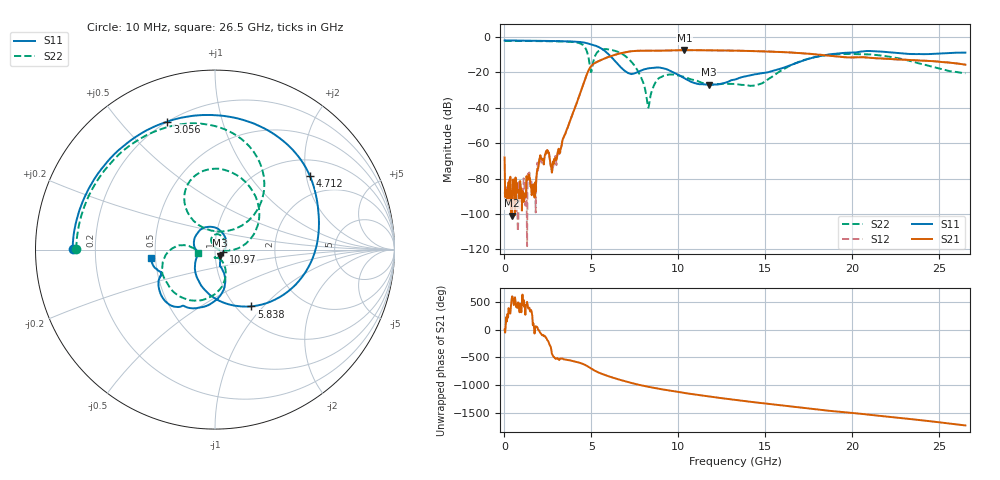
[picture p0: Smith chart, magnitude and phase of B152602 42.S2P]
!  2-Port S-parameters saved by WinCal
! VAR MeasName=S-Parameters (CALIBRATED_DATA) read from VNA (N5242A)
! VAR MeasDate=2016-1-5 16:32:14
! VAR NAME=B152602 42
! VAR FILENAME=B152602 42.S2P
! VAR DATE=2016-1-5 16:32:14
! VAR PHYS_PORTS=1,2
# Hz S DB R 50
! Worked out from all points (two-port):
!   801 points, 10 MHz to 26.5 GHz, reference 50 ohm
!   highest |S21| = -7.47 dB at 10.34 GHz (marker M1); lowest = -100.9 dB at 440.5 MHz (marker M2)
!   |S21| within 3 dB of the highest: 6.238 GHz to 18.54 GHz (12.3 GHz wide, 99.3 % of centre)
!   lowest |S11| = -27.1 dB at 11.73 GHz (marker M3), VSWR 1.09, Z = 52.9 - j3.53 ohm
!   |S11| at or under -10 dB: 6.005 GHz to 18.63 GHz (12.62 GHz wide, 102 % of centre)
!   |S22| runs from -39.9 to -2.2 dB; largest |S21 - S12| = 0.0031
!   S11 on the Smith chart (normalised r, x): 10 MHz: 0.12, +0.00; 3.056 GHz: 0.20, +0.68; 4.712 GHz: 1.41, +2.10; 5.838 GHz: 1.17, -0.86; 10.97 GHz: 1.10, -0.03; 26.5 GHz: 0.47, -0.05
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1e7  -2.01 179.7  -68.07 0.8  -88.54 20.5  -2.23 179.8
4.404625e8  -2.04 170.9  -100.94 -124.4  -86.64 126.1  -2.25 173.2
1.698738e9  -2.20 144.7  -84.91 45.0  -89.84 24.8  -2.36 153.3
2.427212e9  -2.28 127.7  -65.81 -160.7  -64.42 -162.4  -2.44 140.5
2.758338e9  -2.32 118.9  -72.60 -89.8  -76.01 -110.0  -2.47 134.0
3.05635e9  -2.37 110.4  -65.44 -151.4  -66.65 -154.8  -2.53 127.5
4.447075e9  -3.00 54.0  -29.22 112.2  -29.24 112.3  -4.14 74.1
4.711975e9  -3.49 37.9  -21.80 74.6  -21.82 74.8  -7.47 49.9
5.009988e9  -4.31 18.4  -16.24 15.7  -16.25 15.9  -19.29 101.8
5.8378e9  -8.50 -57.3  -11.89 -100.6  -11.86 -100.6  -6.92 87.6
6.6325e9  -16.60 -139.2  -9.35 -179.4  -9.34 -179.5  -8.93 48.8
7.360975e9  -20.89 -169.4  -8.03 118.4  -8.03 118.4  -14.76 12.5
8.255012e9  -17.81 154.1  -7.83 55.3  -7.82 55.2  -39.82 42.9
8.851038e9  -17.25 120.0  -7.83 20.7  -7.84 20.6  -23.57 107.9
1.03411e10  -23.31 21.8  -7.47 -55.6  -7.47 -55.6  -22.63 45.6
1.097024e10  -26.16 -16.4  -7.50 -85.0  -7.49 -84.9  -24.52 15.6
1.173182e10  -27.06 -48.8  -7.57 -118.2  -7.56 -118.1  -26.71 -27.7
1.3255e10  -24.04 -63.1  -7.78 -179.8  -7.78 -179.8  -26.55 -89.1
1.540731e10  -19.27 -70.8  -8.34 98.8  -8.30 98.8  -22.38 -58.3
1.769208e10  -11.83 -83.1  -9.68 16.6  -9.64 16.7  -11.77 -93.2
2.209604e10  -8.64 -148.4  -12.46 -123.1  -12.41 -123.6  -11.12 -173.1
2.65e10  -8.89 -172.8  -15.69 81.7  -15.71 81.4  -20.54 -168.5
